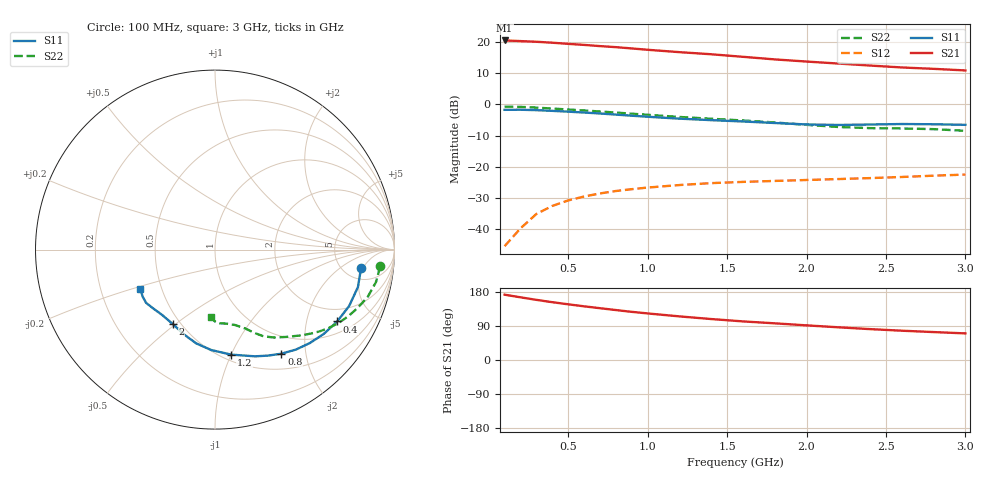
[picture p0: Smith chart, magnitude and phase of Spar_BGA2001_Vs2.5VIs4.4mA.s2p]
! Filename: 2_5G1.001
! Title: BGA2001 X0297-20 HFE=80
! Bias: Vce=2.5V,Ic=4.4mA
! Company: NXP Semiconductors NL
! User: Quality&Reliability T&D
! Measure time: 23 Oct 1998 / 09:19:57
#  MHz  S  MA  R 50
! Freq  S11  S21  S12  S22  :
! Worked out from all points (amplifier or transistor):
!   20 points, 100 MHz to 3 GHz, reference 50 ohm
!   highest |S21| = 20.6 dB at 100 MHz (marker M1)
!   |S21| within 3 dB of that: start of sweep to 1.001 GHz
!   unconditionally stable (mu >= 1): 2.082 GHz to end of sweep
!   at 400 MHz: K = 0.22, MSG = 26.3 dB, |S12| = -32.7 dB
!   at 1.2 GHz: K = 0.55, MSG = 21.4 dB, |S12| = -25.9 dB
!   at 3 GHz: K = 1.23, MAG = 13.9 dB, |S12| = -22.6 dB
!   S11 on the Smith chart (normalised r, x): 100 MHz: 7.26, -4.53; 400 MHz: 1.43, -3.05; 800 MHz: 0.72, -1.58; 1.2 GHz: 0.55, -1.00; 2 GHz: 0.46, -0.49; 3 GHz: 0.38, -0.21
100  0.8202 -7.2  10.73 172.3  0.005248 58.5  0.9255 -5.8
200  0.8233 -14.7  10.48 165.4  0.01015 80.6  0.915 -11.4
300  0.8107 -22.8  10.22 158.7  0.01732 78.9  0.8913 -17.1
400  0.7898 -30.5  9.866 152.6  0.0233 74.2  0.86 -22.0
500  0.7672 -37.6  9.451 146.9  0.02857 70.2  0.8308 -26.5
600  0.742 -44.5  9.1 141.7  0.03305 66.6  0.801 -30.6
700  0.7165 -51.0  8.705 136.7  0.03701 63.5  0.7717 -34.3
800  0.6878 -57.5  8.374 131.8  0.04052 60.6  0.7415 -37.8
900  0.6599 -63.5  7.979 127.0  0.04335 58.3  0.7114 -41.1
1000  0.6347 -69.5  7.597 122.9  0.04604 56.4  0.6825 -44.3
1200  0.5918 -81.3  6.953 115.1  0.05054 53.1  0.6301 -50.5
1400  0.5598 -92.2  6.431 108.1  0.05427 50.7  0.5894 -56.2
1600  0.533 -101.3  5.852 101.9  0.05679 49.6  0.553 -60.8
1800  0.5036 -109.9  5.316 96.8  0.05887 49.9  0.5139 -64.6
2000  0.4774 -119.3  4.909 91.4  0.06095 49.3  0.4705 -69.0
2200  0.4683 -129.0  4.559 86.3  0.06309 48.9  0.4346 -75.1
2400  0.4761 -136.9  4.233 81.5  0.06538 49.3  0.4163 -81.8
2600  0.4851 -142.3  3.944 77.3  0.06814 50.9  0.4116 -86.8
2800  0.4807 -146.9  3.747 73.7  0.07152 51.4  0.4012 -90.0
3000  0.4706 -152.5  3.531 70.2  0.07447 52.3  0.3768 -93.3
